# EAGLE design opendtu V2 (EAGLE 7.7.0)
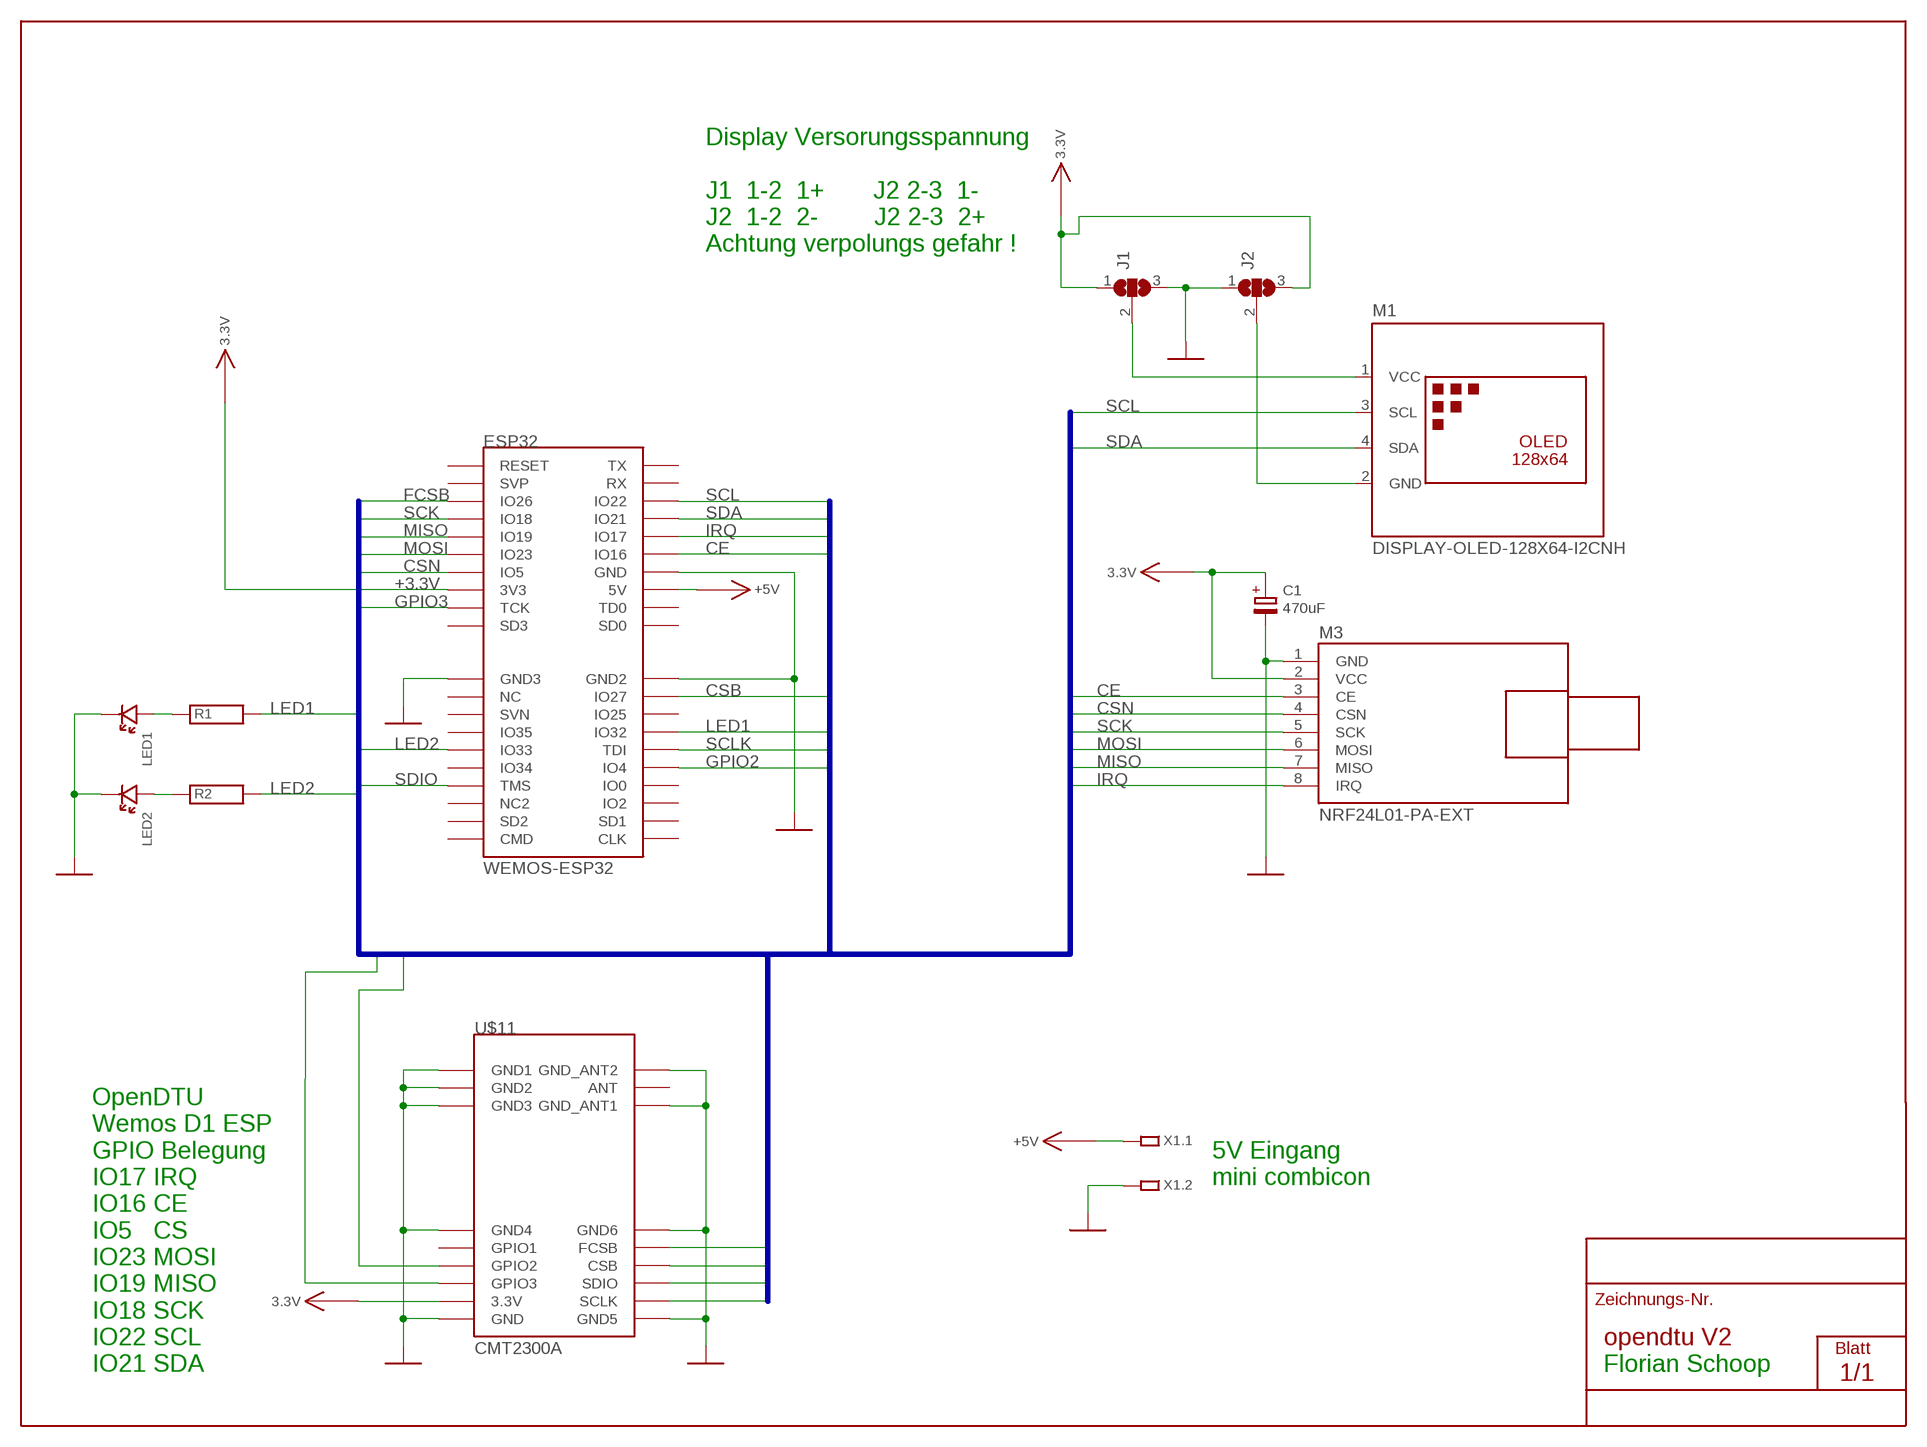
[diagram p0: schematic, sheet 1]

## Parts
C1  470uF  S470µ/16  [EB10D]
ESP32  WEMOS-ESP32  [WEMOS-ESP32]
J1  SJ2W  [SJ_2]
J2  SJ2W  [SJ_2]
LED1  LED3MM  [LED3MM]
LED2  LED3MM  [LED3MM]
M1  DISPLAY-OLED-128X64-I2CNH  [DISPLAY-OLED-128X64-I2C_NH]
M3  NRF24L01-PA-EXT  [NRF24L01-PA-EXT]
R1  WIDERSAND  [1/8W]
R2  WIDERSAND  [1/8W]
U$11  CMT2300A  [CMT2300A]
X1  MCV1,5/2G  [MCV1,5/2]

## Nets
+3.3V: C1.+ ESP32.3V3 J1.1 J2.3 M3.2(VCC) U$11.3.3V ; supply symbol labelled 3.3V
+5V: ESP32.VCC(5V) X1.1
CE: ESP32.IO16 M3.3(CE)
CSB: ESP32.IO27 U$11.CSB
CSN: ESP32.IO5 M3.4(CSN)
FCSB: ESP32.IO26 U$11.FCSB
GND: C1.- ESP32.GND ESP32.GND2 ESP32.GND3 J1.3 J2.1 LED1.K(KAT) LED2.K(KAT) M3.1(GND) U$11.GND U$11.GND1 U$11.GND2 U$11.GND3 U$11.GND4 U$11.GND5 U$11.GND6 U$11.GND_ANT1 U$11.GND_ANT2 X1.2
GPIO2: ESP32.IO4 U$11.GPIO2
GPIO3: ESP32.TCK U$11.GPIO3
IRQ: ESP32.IO17 M3.8(IRQ)
LED1: ESP32.IO32 R1.2
LED2: ESP32.IO33 R2.2
MISO: ESP32.IO19 M3.7(MISO)
MOSI: ESP32.IO23 M3.6(MOSI)
N$3: J2.2 M1.2(GND)
N$4: J1.2 M1.1(VCC)
N$5: LED2.A(ANO) R2.1
N$6: LED1.A(ANO) R1.1
SCK: ESP32.IO18 M3.5(SCK)
SCL: ESP32.IO22 M1.3(SCL)
SCLK: ESP32.TDI U$11.SCLK
SDA: ESP32.IO21 M1.4(SDA)
SDIO: ESP32.TMS U$11.SDIO
Unconnected: ESP32.CLK ESP32.CMD ESP32.IO0 ESP32.IO2 ESP32.IO25 ESP32.IO34 ESP32.IO35 ESP32.NC ESP32.NC1(NC2) ESP32.RST(RESET) ESP32.RXD(RX) ESP32.SD0 ESP32.SD1 ESP32.SD2 ESP32.SD3 ESP32.SVN ESP32.SVP ESP32.TD0 ESP32.TXD(TX) U$11.ANT U$11.GPIO1

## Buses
B$1

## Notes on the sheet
- Display Versorungsspannung
  
  J1  1-2  1+       J2 2-3  1-
  J2  1-2  2-        J2 2-3  2+
  Achtung verpolungs gefahr !
- 5V Eingang
  mini combicon
- OpenDTU 
  Wemos D1 ESP
  GPIO Belegung
  IO17 IRQ
  IO16 CE
  IO5   CS
  IO23 MOSI
  IO19 MISO
  IO18 SCK
  IO22 SCL
  IO21 SDA
- Florian Schoop

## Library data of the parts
C1 = 5elko:S470µ/16
ESP32 = wemos d1:WEMOS-ESP32
J1 J2 = jumper_fs:SJ2W: SMD solder JUMPER
LED1 LED2 = LED:LED3MM
M1 = EYR_Displays:DISPLAY-OLED-128X64-I2C: 128x64 Dot Matrix OLED Module based on SSD1306 chip Variant with I2C interface
M3 = EYR_Modulos:NRF24L01-PA-EXT: 2.4 GHz Wireless Module based on NRF24L01 chip with preamplifier and external antenna
R1 R2 = 1WIDER:WIDERSAND
U$11 = cmt2300a:CMT2300A
X1 = STECKER:MCV1,5/2G

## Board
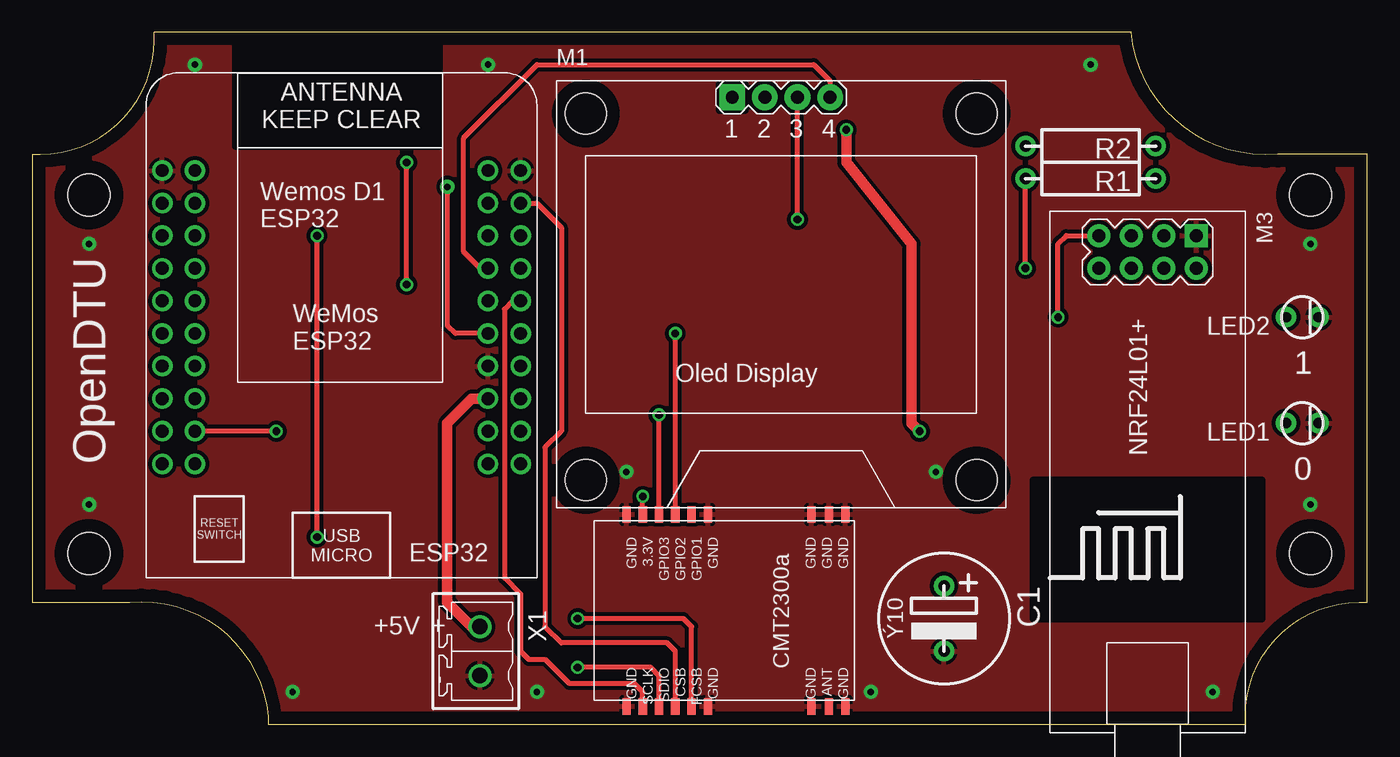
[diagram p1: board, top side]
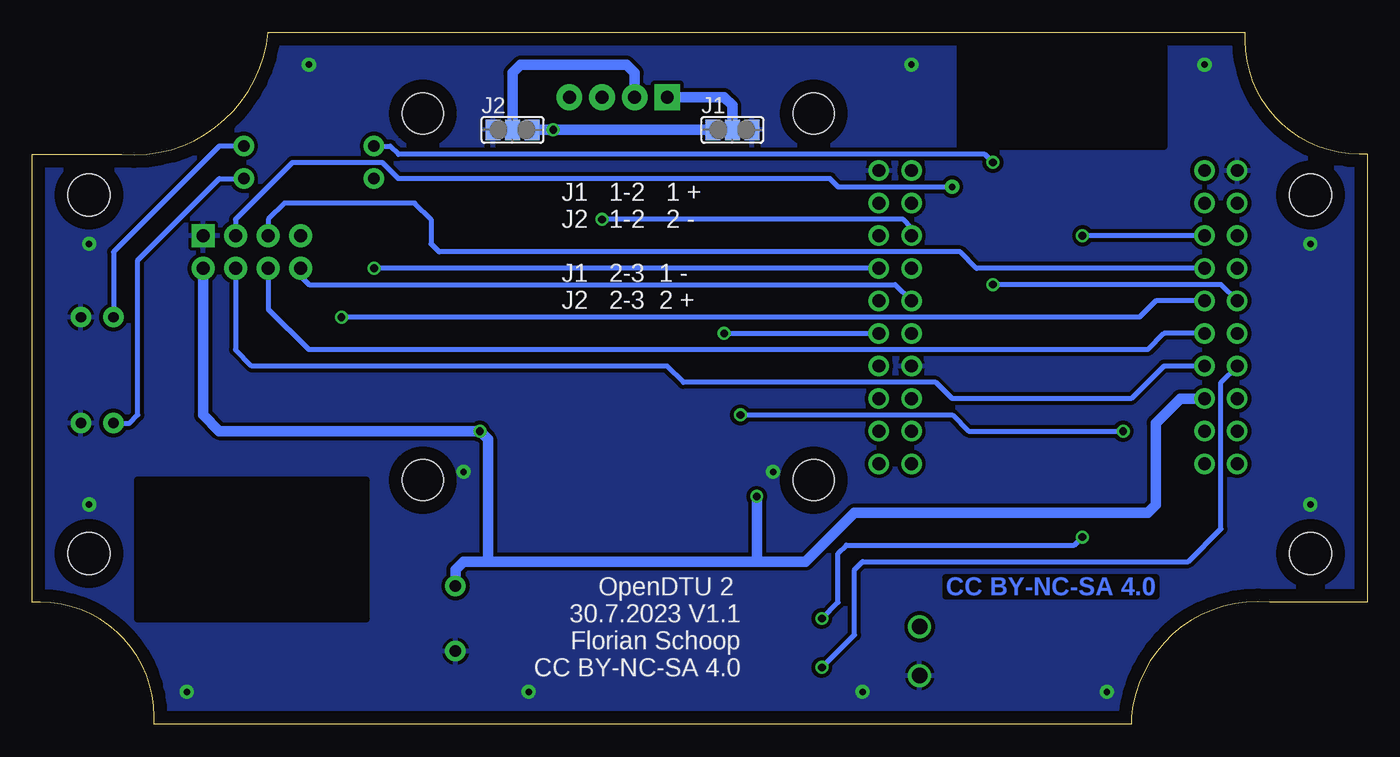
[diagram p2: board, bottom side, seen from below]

Size 104.14 x 53.98 mm. Coordinates in mm from the lower left corner, seen from the top.
Outline: 104.14,9.53 104.14,44.45 97.16,44.45 arc-90 85.72,53.98 9.53,53.98 9.53,53.34 arc-90 0.64,44.45 0,44.45 0,9.53 7.62,9.53 arc-90 18.41,0.64 18.41,0 94.61,0 94.61,0.64 arc-90 103.5,9.53 104.14,9.53
Copper layers (1*16): Component 0.035mm / dielectric 1.5mm / Solder 0.035mm
Design rules "default": minimum track width 10mil, minimum drill 0.6mm, track to track 8mil, track to pad 8mil, pad to pad 8mil, via to via 8mil, smd to smd 8mil, copper to edge 40mil, drill to drill 8mil, minimum pad ring 10mil, minimum via ring 8mil, stop-mask expansion 4mil, vias tented up to drill 0mil, thermal gap 10mil
Holes 3.3 mm at 4.45,41.27 4.45,13.34 99.69,41.27 99.69,13.34
Holes 3.2 mm at 43.18,47.62 73.66,47.62 73.66,19.05 43.18,19.05
tRestrict: area 15.9,45.1 to 31.7,54; area 78.1,8.3 to 95.9,19
bRestrict: area 15.9,45.1 to 31.7,54; area 78.1,8.3 to 95.9,19

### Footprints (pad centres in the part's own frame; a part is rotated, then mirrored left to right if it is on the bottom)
EB10D = drill 0.9 pad 1.6: + -2.54,0; - 2.54,0
WEMOS-ESP32 = drill 1 pad 1.6: 3V3 2.54,11.43; CLK 27.94,6.35; CMD 0,6.35; GND 25.4,13.97; GND2 27.94,29.21; GND3 0,29.21; IO0 27.94,13.97; IO2 27.94,11.43; IO4 27.94,16.51; IO5 2.54,13.97; IO16 25.4,16.51; IO17 25.4,19.05; IO18 2.54,21.59; IO19 2.54,19.05; IO21 25.4,21.59; IO22 25.4,24.13; IO23 2.54,16.51; IO25 27.94,24.13; IO26 2.54,24.13; IO27 27.94,26.67; IO32 27.94,21.59; IO33 0,19.05; IO34 0,16.51; IO35 0,21.59; NC 0,26.67; NC1 0,11.43; RST 2.54,29.21; RXD 25.4,26.67; SD0 25.4,6.35; SD1 27.94,8.89; SD2 0,8.89; SD3 2.54,6.35; SVN 0,24.13; SVP 2.54,26.67; TCK 2.54,8.89; TD0 25.4,8.89; TDI 27.94,19.05; TMS 0,13.97; TXD 25.4,29.21; VCC 25.4,11.43
SJ_2 = smd 1.168 x 1.6: 1 -1.524,0; 2 0,0; 3 1.524,0
LED3MM = drill 0.8 pad 1.6: A 1.27,0; K -1.27,0
DISPLAY-OLED-128X64-I2C_NH = drill 1 pad 2 square: 1 -3.81,12.7 | drill 1 pad 2: 2 -1.27,12.7; 3 1.27,12.7; 4 3.81,12.7
NRF24L01-PA-EXT = drill 1 pad 1.778 square: 1 -18.415,3.81 | drill 1.016 pad 1.778: 2 -15.875,3.81; 3 -18.415,1.27; 4 -15.875,1.27; 5 -18.415,-1.27; 6 -15.875,-1.27; 7 -18.415,-3.81; 8 -15.875,-3.81
1/8W = drill 0.9 pad 1.6: 1 0,0; 2 10.16,0
CMT2300A = smd 1.27 x 0.635: 3.3V -0.5,2.54; ANT 14.47,17.07; CSB 14.47,5.08; FCSB 14.47,6.35; GND -0.5,1.27; GND1 -0.5,18.34; GND2 -0.5,17.07; GND3 -0.5,15.7; GND4 -0.5,7.62; GND5 14.47,1.27; GND6 14.47,7.62; GND_ANT1 14.47,15.7; GND_ANT2 14.47,18.34; GPIO1 -0.5,6.35; GPIO2 -0.5,5.08; GPIO3 -0.5,3.81; SCLK 14.47,2.54; SDIO 14.47,3.81
MCV1,5/2 = drill 1.2 pad 1.6: 1 0,0; 2 3.81,0

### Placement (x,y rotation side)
C1  71.12,8.26 270 top
ESP32  10.16,13.97 0 top
J1  49.53,46.36 0 bottom
J2  66.67,46.36 0 bottom
LED1  99.06,23.49 180 top
LED2  99.06,31.75 180 top
M1  58.42,36.2 0 top
M3  86.99,19.68 270 top
R1  87.63,42.55 180 top
R2  87.63,45.09 180 top
U$11  45.09,15.88 270 top
X1  34.93,7.62 270 top

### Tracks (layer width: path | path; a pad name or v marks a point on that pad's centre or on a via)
+3.3V  (via drill 0.6)
  Component 0.406: U$11.3.3V v47.62,17.78
  Component 0.813: v69.21,22.86 68.58,23.49 68.58,37.47 63.5,43.82 v63.5,46.36
  Solder 0.406: 65.41,46.36 J2.3
  Solder 0.813: J1.1 v63.5,46.36 J2.3 | ESP32.3V3 14.61,25.4 16.51,23.49 16.51,17.14 17.14,16.51 40.01,16.51 43.82,12.7 47.62,12.7 | 68.58,12.7 68.58,22.22 v69.21,22.86 89.53,22.86 90.8,24.13 M3.2 | v47.62,17.78 47.62,12.7 | 47.62,12.7 68.58,12.7 | 68.58,12.7 70.48,12.7 71.12,12.06 C1.+
+5V
  Component 0.813: X1.1 34.29,7.62 32.39,9.53 32.39,23.49 34.29,25.4 ESP32.VCC
CE  (via drill 0.5 pad 1.1)
  Component 0.406: v32.39,41.91 32.39,31.11 33.02,30.48 ESP32.IO16
  Solder 0.406: v32.39,41.91 41.27,41.91 41.91,42.55 75.56,42.55 76.83,43.82 83.82,43.82 88.27,39.37 M3.3
CSB
  Component 0.406: ESP32.IO27 39.37,40.64 41.27,38.73 41.27,22.86 40.01,21.59 40.01,7.62 41.27,6.35 49.53,6.35 50.16,5.71 U$11.CSB
CSN
  Solder 0.406: ESP32.IO5 15.88,27.94 18.41,25.4 32.39,25.4 33.66,26.67 53.34,26.67 54.61,27.94 86.99,27.94 88.27,29.21 M3.4
FCSB  (via drill 0.6)
  Component 0.406: U$11.FCSB 51.44,7.62 50.8,8.26 v42.55,8.26 | v22.22,14.61 v22.22,38.1
  Solder 0.406: v42.55,8.26 41.27,9.53 41.27,13.34 40.64,13.97 22.86,13.97 v22.22,14.61 | ESP32.IO26 v22.22,38.1
GND  (via drill 0.5 pad 1.1)
  other vias: 46.36,19.68 70.48,19.68 12.7,51.44 82.55,51.44 20.32,2.54 92.07,2.54 4.45,17.14 4.45,37.47 35.56,51.44 99.69,37.47 99.69,17.14 65.41,2.54 39.37,2.54
  pour Component (isolate 0.3): 9.53,53.98 85.72,53.98 arc90 95.25,44.45 96.52,44.45 104.14,44.45 104.14,31.75 104.14,9.53 arc90 94.61,0 73.02,0 18.41,0 arc90 8.89,9.53 5.08,9.53 0,9.53 0,12.06 0,44.45 arc90
  pour Solder (isolate 0.3): 9.53,53.98 85.72,53.98 arc90 95.25,44.45 104.14,44.45 104.14,9.53 arc90 94.61,0 59.05,0 18.41,0 arc90 8.89,9.53 0,9.53 0,26.04 0,44.45 arc90
GPIO2  (via drill 0.6)
  Component 0.406: U$11.GPIO2 v50.16,30.48
  Solder 0.406: v50.16,30.48 ESP32.IO4
GPIO3  (via drill 0.6)
  Component 0.406: U$11.GPIO3 v48.9,24.13 | v19.05,22.86 ESP32.TCK
  Solder 0.406: v48.9,24.13 32.39,24.13 31.11,22.86 v19.05,22.86
IRQ
  Solder 0.406: ESP32.IO17 36.83,34.29 82.55,34.29 83.18,34.93 M3.8
LED1  (via drill 0.6)
  Component 0.406: v77.47,35.56 R1.2
  Solder 0.406: ESP32.IO32 v77.47,35.56
LED2  (via drill 0.6)
  Component 0.406: v29.21,34.29 v29.21,43.82
  Solder 0.406: ESP32.IO33 11.43,34.29 v29.21,34.29 | v29.21,43.82 29.84,44.45 75.56,44.45 76.2,45.09 R2.2
MISO  (via drill 0.6)
  Component 0.406: v80.01,31.75 80.01,37.47 80.64,38.1 M3.7
  Solder 0.406: ESP32.IO19 16.51,33.02 17.78,31.75 v80.01,31.75
MOSI
  Solder 0.406: ESP32.IO23 15.88,30.48 17.14,29.21 82.55,29.21 85.72,32.39 M3.6
N$3
  Solder 0.813: M1.2 57.15,50.8 57.79,51.44 66.04,51.44 66.67,50.8 J2.2
N$4
  Solder 0.813: J1.2 49.53,48.26 50.16,48.9 M1.1
N$5
  Solder 0.406: R2.1 89.53,45.09 97.79,36.83 LED2.A
N$6
  Solder 0.406: LED1.A 96.52,23.49 95.88,24.13 95.88,36.2 89.53,42.55 R1.1
SCK
  Solder 0.406: ESP32.IO18 30.48,35.56 31.75,36.83 72.39,36.83 73.02,37.47 73.02,39.37 74.3,40.64 84.45,40.64 85.72,39.37 M3.5
SCL  (via drill 0.6)
  Component 0.406: v59.69,39.37 M1.3
  Solder 0.406: v59.69,39.37 36.2,39.37 35.56,38.73 ESP32.IO22
SCLK
  Component 0.406: U$11.SCLK 47.62,2.54 46.99,3.17 41.91,3.17 40.01,5.08 38.73,5.08 38.1,5.71 38.1,10.16 36.83,11.43 36.83,32.39 37.47,33.02 ESP32.TDI
SDA
  Component 0.406: ESP32.IO21 34.93,35.56 33.66,36.83 33.66,45.72 39.37,51.44 60.96,51.44 62.23,50.16 M1.4
SDIO  (via drill 0.6)
  Component 0.406: U$11.SDIO 48.9,3.81 48.26,4.45 v42.55,4.45
  Solder 0.406: v42.55,4.45 40.01,6.99 40.01,12.06 39.37,12.7 13.97,12.7 11.43,15.24 11.43,26.67 ESP32.TMS

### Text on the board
Solder: CC BY-NC-SA 4.0
tNames: 1 | 2 | 3 | 4 | Wemos D1 / ESP32 | 1 | Oled Display | NRF24L01+ | OpenDTU | 0 | +5V | + | -
bNames: J1 1-2 1 + / J2 1-2 2 - / / J1 2-3 1 - / J2 2-3 2 + | OpenDTU 2 / 30.7.2023 V1.1 / Florian Schoop / CC BY-NC-SA 4.0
